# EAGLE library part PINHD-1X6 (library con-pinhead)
PIN HEADER
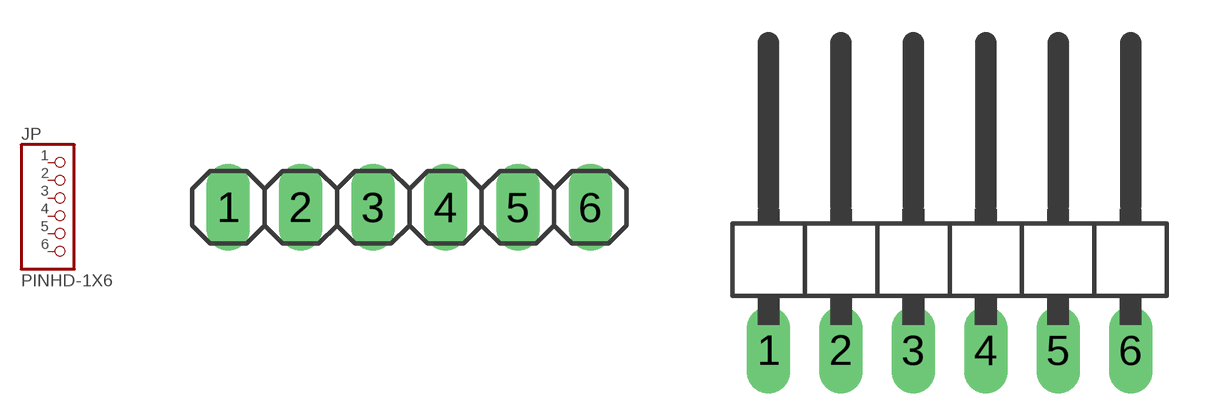
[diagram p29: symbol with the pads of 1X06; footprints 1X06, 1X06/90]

Designator prefix JP

## PINHD-1X6_2.54  [1X06]
1  1  pas
2  2  pas
3  3  pas
4  4  pas
5  5  pas
6  6  pas

## PINHD-1X6_2.54-90°  [1X06/90]
Pads as for 1X06

## PINHD-1X6_2.00  [1X06M]
Pads as for 1X06

## PINHD-1X6_2.54-SMD  [1X06SMD]
Pads as for 1X06

## PINHD-1X6_2.54-SMD-90°  [1X06SMD/90]
Pads as for 1X06

## Footprint 1X06 (pad centres in mm)
PIN HEADER - 2.54
drill 1.016 long: 1 -6.35,0; 2 -3.81,0; 3 -1.27,0; 4 1.27,0; 5 3.81,0; 6 6.35,0

## Footprint 1X06/90 (pad centres in mm)
PIN HEADER - 2.54 90°
drill 1.016 long: 1 -6.35,-3.81; 2 -3.81,-3.81; 3 -1.27,-3.81; 4 1.27,-3.81; 5 3.81,-3.81; 6 6.35,-3.81

## Footprint 1X06M (pad centres in mm)
PIN HEADER - 2
drill 0.914 square: 1 -5,0
drill 0.914: 2 -3,0; 3 -1,0; 4 1,0; 5 3,0; 6 5,0

## Footprint 1X06SMD (pad centres in mm)
PIN HEADER - 2.54 SMD
smd 1.016 x 3.302: 1 -1.27,1.27; 2 1.27,-1.27; 3 3.81,1.27; 4 6.35,-1.27; 5 8.89,1.27; 6 11.43,-1.27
